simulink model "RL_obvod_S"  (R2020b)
settings: Solver=VariableStepAuto  StartTime=0.0  StopTime=Tsim  MaxStep=1e-5  RelTol=1e-8
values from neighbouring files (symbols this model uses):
  L = 10e-3    (= 0.01)    [RL_obvod_M.m]
  R = 10    [RL_obvod_M.m]
  w = 1500    [RL_obvod_M.m]
libraries: simulink x1

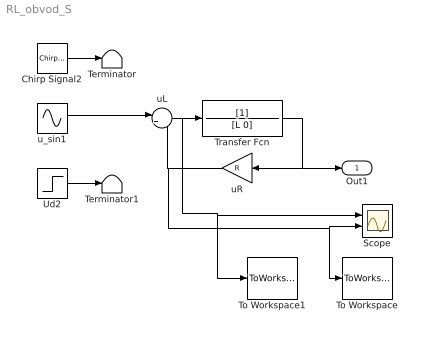
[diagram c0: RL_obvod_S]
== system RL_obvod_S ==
  Chirp Signal2 : simulink/Sources/Chirp Signal  f1=1/(2*pi)  T=.05  f2=1e5/(2*pi)
  Scope : Scope  NumInputPorts=2
  Terminator : Terminator
  Terminator1 : Terminator
  To Workspace : ToWorkspace  VariableName=uR  SampleTime=-1
  To Workspace1 : ToWorkspace  VariableName=uL  SampleTime=-1
  Transfer Fcn : TransferFcn  Denominator=[L 0]
  Ud2 : Step  Time=0  SampleTime=0
  uL : Sum  Inputs=|+-
  uR : Gain  Gain=R
  u_sin1 : Sin  Frequency=w  SampleTime=0
  Out1 : Outport
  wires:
  Transfer Fcn/1 -> uR/1, Out1/1
  Chirp Signal2/1 -> Terminator/1
  Ud2/1 -> Terminator1/1
  uL/1 -> To Workspace1/1, Scope/1, Transfer Fcn/1
  uR/1 -> To Workspace/1, Scope/2, uL/2
  u_sin1/1 -> uL/1
